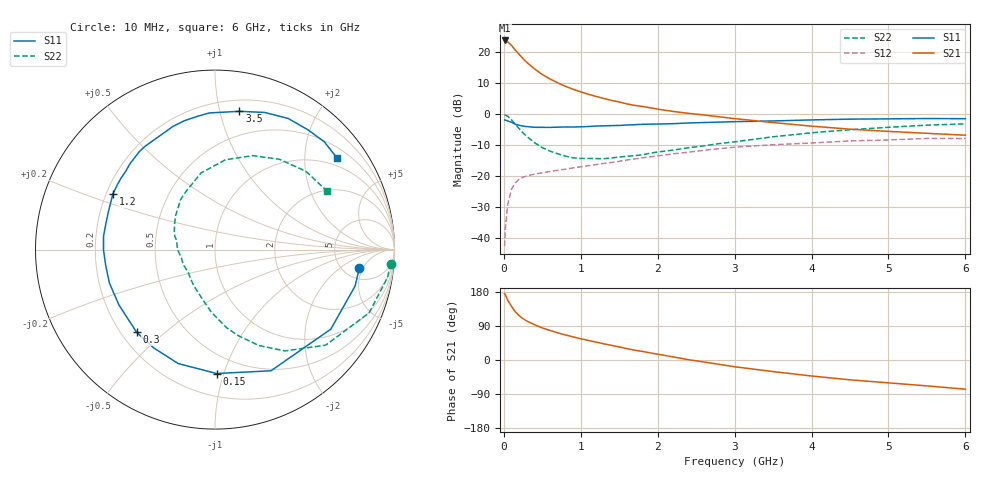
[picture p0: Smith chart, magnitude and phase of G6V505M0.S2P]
! SIEMENS Small Signal Semiconductors
! BFG193
! Si NPN RF Bipolar Junction Transistor in SOT223
! VCE = 0.5 V  IC = 5 mA
! Common Emitter S-Parameters:  August  1996
# GHz  S  MA  R  50
!  f  S11  S21  S12  S22
! GHz  MAG  ANG  MAG  ANG  MAG  ANG  MAG  ANG
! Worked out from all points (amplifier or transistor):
!   36 points, 10 MHz to 6 GHz, reference 50 ohm
!   highest |S21| = 23.8 dB at 10 MHz (marker M1)
!   |S21| within 3 dB of that: start of sweep to 145.4 MHz
!   unconditionally stable (mu >= 1): 997.9 MHz to 4.465 GHz; 4.609 GHz to 5.229 GHz; 5.662 GHz to end of sweep
!   at 250 MHz: K = 0.36, MSG = 19.1 dB, |S12| = -20.3 dB
!   at 1.4 GHz: K = 1.12, MAG = 7.9 dB, |S12| = -15.5 dB
!   at 6 GHz: K = 1.01, MAG = -0.2 dB, |S12| = -7.8 dB
!   S11 on the Smith chart (normalised r, x): 10 MHz: 7.11, -4.16; 150 MHz: 0.36, -0.95; 300 MHz: 0.26, -0.40; 1.2 GHz: 0.23, +0.24; 3.5 GHz: 0.29, +1.15; 6 GHz: 0.77, +2.82
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0.01  0.8109 -7.1  15.51 175.5  0.0075 87.0  0.9816 -4.6
0.02  0.8065 -14.6  15.38 171.9  0.0146 81.8  0.9736 -9.2
0.05  0.7827 -34.5  14.72 158.0  0.0355 72.1  0.9283 -22.3
0.1  0.7437 -65.2  12.91 141.5  0.0623 58.9  0.8147 -40.8
0.15  0.6906 -89.2  10.8 126.8  0.0792 47.9  0.6861 -55.4
0.2  0.6672 -107.9  9.231 117.1  0.0898 41.9  0.5877 -65.4
0.25  0.6455 -122.0  7.883 108.9  0.0971 37.0  0.4999 -74.5
0.3  0.6346 -133.5  6.838 102.7  0.1018 34.5  0.4399 -81.6
0.4  0.6178 -150.0  5.376 93.0  0.109 30.6  0.3481 -93.5
0.5  0.6171 -162.6  4.381 84.7  0.1142 28.6  0.2899 -103.1
0.6  0.6154 -172.0  3.719 78.0  0.12 28.2  0.2555 -112.0
0.8  0.6256 173.2  2.828 66.2  0.1308 27.6  0.2124 -129.7
0.9  0.6247 167.1  2.537 61.1  0.1372 27.6  0.199 -137.3
1.1  0.6367 156.2  2.102 51.6  0.1485 27.2  0.1945 -152.1
1.2  0.6478 151.4  1.941 47.2  0.1551 27.1  0.1935 -159.2
1.6  0.6736 134.6  1.472 30.0  0.1837 24.3  0.2107 176.4
2.2  0.707 114.8  1.113 8.2  0.2304 16.9  0.2652 148.3
2.8  0.749 97.5  0.911 -11.5  0.28 6.5  0.3379 124.7
3.5  0.7823 80.0  0.736 -30.6  0.3238 -8.9  0.4344 100.3
4.5  0.8367 60.8  0.576 -52.3  0.3725 -27.3  0.5642 68.1
5.5  0.8553 44.6  0.494 -68.3  0.4083 -49.5  0.6687 40.7
6  0.8501 36.8  0.461 -77.1  0.4075 -62.2  0.703 27.8
